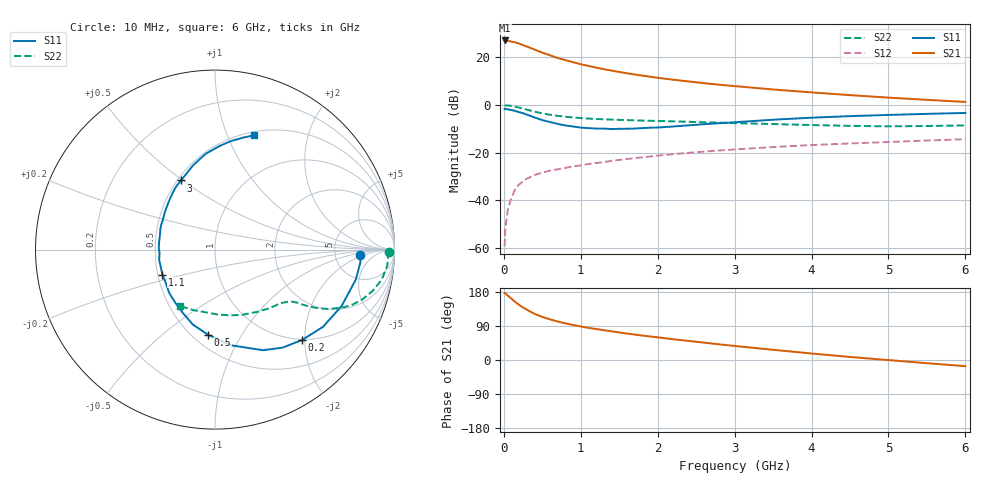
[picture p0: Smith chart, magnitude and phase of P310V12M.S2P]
! SIEMENS Small Signal Semiconductors
! BFP181
! Si NPN RF Bipolar Junction Transistor in SOT143
! VCE = 10 V  IC = 12 mA
! Common Emitter S-Parameters:  March  1996
# GHz  S  MA  R  50
!  f  S11  S21  S12  S22
! GHz  MAG  ANG  MAG  ANG  MAG  ANG  MAG  ANG
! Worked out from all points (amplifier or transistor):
!   36 points, 10 MHz to 6 GHz, reference 50 ohm
!   highest |S21| = 26.9 dB at 10 MHz (marker M1)
!   |S21| within 3 dB of that: start of sweep to 335.7 MHz
!   unconditionally stable (mu >= 1): 1.287 GHz to end of sweep
!   at 250 MHz: K = 0.34, MSG = 28.5 dB, |S12| = -32.1 dB
!   at 1.4 GHz: K = 1.03, MAG = 17.9 dB, |S12| = -23.5 dB
!   at 6 GHz: K = 1.04, MAG = 6.6 dB, |S12| = -14.4 dB
!   S11 on the Smith chart (normalised r, x): 10 MHz: 9.19, -1.74; 200 MHz: 0.98, -1.94; 500 MHz: 0.59, -0.73; 1.1 GHz: 0.53, -0.16; 3 GHz: 0.52, +0.49; 6 GHz: 0.54, +1.25
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0.01  0.81 -2.3  22.09 176.6  0.0011 71.2  0.9701 -0.7
0.02  0.8134 -4.9  21.92 175.6  0.0026 73.6  0.9654 -1.9
0.05  0.8021 -12.0  21.79 170.3  0.0061 85.7  0.964 -5.3
0.1  0.7723 -24.0  20.88 161.5  0.0117 75.9  0.9439 -10.3
0.15  0.7397 -35.6  20.11 152.8  0.0172 70.7  0.9076 -14.7
0.2  0.699 -46.1  19.02 145.2  0.0216 67.6  0.8676 -18.6
0.25  0.6635 -55.4  17.58 138.4  0.0249 63.0  0.8255 -21.8
0.3  0.6211 -64.5  16.47 132.7  0.0286 60.2  0.7874 -24.1
0.4  0.5406 -80.5  14.24 121.7  0.0338 56.1  0.7146 -27.6
0.5  0.4763 -94.6  12.26 113.7  0.0381 53.1  0.6587 -29.7
0.6  0.4356 -106.4  10.81 107.2  0.0418 51.7  0.6174 -31.0
0.7  0.3964 -116.7  9.499 101.6  0.0445 50.8  0.5849 -31.9
0.9  0.3506 -136.9  7.758 92.5  0.0511 49.8  0.5409 -33.0
1.1  0.3242 -154.6  6.493 84.8  0.0575 49.7  0.5133 -34.3
1.3  0.3167 -169.4  5.531 78.6  0.0634 49.1  0.4954 -36.0
1.6  0.3145 171.3  4.56 69.9  0.0732 48.4  0.477 -38.6
2.2  0.3504 142.6  3.336 54.8  0.0922 45.6  0.4482 -46.1
3  0.4293 116.2  2.45 37.1  0.116 39.9  0.4119 -58.3
3.5  0.4855 104.5  2.085 26.9  0.1302 35.9  0.3941 -67.3
4.5  0.5771 87.6  1.586 8.0  0.1548 27.7  0.3613 -88.2
5.5  0.6438 75.8  1.264 -8.5  0.1784 20.5  0.3585 -110.4
6  0.6733 71.1  1.143 -16.2  0.1897 16.5  0.3692 -121.8
